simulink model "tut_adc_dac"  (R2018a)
settings: Solver=VariableStepAuto  StartTime=0.0  StopTime=10.0  RelTol=1e-3
undefined symbols (not defined in the file): adc_data_ch1, adc_data_ch2, adc_data_valid, Bit, Both, bram, c, d, hex2dec, led, Location, Lower, Minimum_Area, out, RED_PITAYA_10, reg, ROACH, ROACH2, rst_cntrl, Unsigned, Upper, Width, xc7z010
libraries: xbsIndex_r4 x149, xps_library x6, casper_library_misc x2
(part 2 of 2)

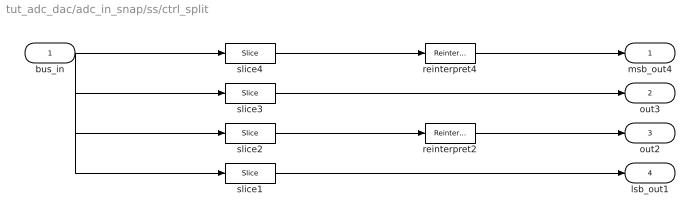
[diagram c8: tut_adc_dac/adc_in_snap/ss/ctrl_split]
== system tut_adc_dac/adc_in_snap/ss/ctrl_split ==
  bus_in : Inport
  reinterpret2 : xbsIndex_r4/Reinterpret  force_arith_type=on  arith_type=Unsigned  force_bin_pt=on  bin_pt=0  block_type=reinterpret
  reinterpret4 : xbsIndex_r4/Reinterpret  force_arith_type=on  arith_type=Unsigned  force_bin_pt=on  bin_pt=0  block_type=reinterpret
  slice1 : xbsIndex_r4/Slice  nbits=1  boolean_output=on  mode=Upper Bit Location + Width  bit1=-31  base1=MSB of Input  bit0=0  base0=LSB of Input  dbl_ovrd=off  block_type=slice
  slice2 : xbsIndex_r4/Slice  nbits=2  boolean_output=off  mode=Upper Bit Location + Width  bit1=-29  base1=MSB of Input  bit0=0  base0=LSB of Input  dbl_ovrd=off  block_type=slice
  slice3 : xbsIndex_r4/Slice  nbits=1  boolean_output=on  mode=Upper Bit Location + Width  bit1=-28  base1=MSB of Input  bit0=0  base0=LSB of Input  dbl_ovrd=off  block_type=slice
  slice4 : xbsIndex_r4/Slice  nbits=28  boolean_output=off  mode=Upper Bit Location + Width  bit1=0  base1=MSB of Input  bit0=0  base0=LSB of Input  dbl_ovrd=off  block_type=slice
  msb_out4 : Outport
  out3 : Outport  Port=2
  out2 : Outport  Port=3
  lsb_out1 : Outport  Port=4
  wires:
  bus_in/1 -> slice4/1, slice3/1, slice2/1, slice1/1
  slice4/1 -> reinterpret4/1
  reinterpret4/1 -> msb_out4/1
  slice3/1 -> out3/1
  slice2/1 -> reinterpret2/1
  reinterpret2/1 -> out2/1
  slice1/1 -> lsb_out1/1

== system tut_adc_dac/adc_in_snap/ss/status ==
  out_reg : Inport
  assert_reg : xbsIndex_r4/Assert  assert_type=on  type_source=Explicitly  gui_display_data_type=Fixed-point  arith_type=Unsigned  n_bits=32  bin_pt=0  preci_type=Single  exp_width=8  frac_width=24  assert_rate=off  rate_source=Explicitly  period=1  output_port=on  block_type=assert
  cast_gw : xbsIndex_r4/Convert  gui_display_data_type=Fixed-point  arith_type=Unsigned  n_bits=32  bin_pt=0  float_type=Single  exp_bits=8  fraction_bits=24  quantization=Truncate  overflow=Wrap  en=off  latency=1  pipeline=off  dbl_ovrd=off  block_type=convert
  io_delay : xbsIndex_r4/Delay  rst=off  infoeditControl=Selection of Reset will increase slice count due to use of real FFs and instead of SRLs  en=off  latency=0  reg_retiming=on  dbl_ovrd=off  block_type=delay
  reint1 : xbsIndex_r4/Reinterpret  force_arith_type=on  arith_type=Unsigned  force_bin_pt=on  bin_pt=0  block_type=reinterpret
  sim_out : Terminator
  tut_adc_dac_adc_in_snap_ss_status_user_data_in : xbsIndex_r4/Gateway Out  inherit_from_input=off  hdl_port=on  rows=1  columns=1  UseAsDAC=off  DACChannel='1'  interface=None  automatic_assignment=on  address_offset=hex2dec('00')  intf_name=''  intf_description=''  timing_constraint=None  locs_specified=off  LOCs={}  io_standard={}  block_type=gatewayout
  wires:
  io_delay/1 -> cast_gw/1
  cast_gw/1 -> tut_adc_dac_adc_in_snap_ss_status_user_data_in/1
  tut_adc_dac_adc_in_snap_ss_status_user_data_in/1 -> sim_out/1
  out_reg/1 -> assert_reg/1
  assert_reg/1 -> reint1/1
  reint1/1 -> io_delay/1

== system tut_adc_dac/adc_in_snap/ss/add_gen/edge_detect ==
  in : Inport
  Delay : xbsIndex_r4/Delay  rst=off  infoeditControl=Selection of Reset will increase slice count due to use of real FFs and instead of SRLs  en=off  latency=1  reg_retiming=off  dbl_ovrd=off  block_type=delay
  Inverter : xbsIndex_r4/Inverter  en=off  latency=0  dbl_ovrd=off  block_type=inv
  edge_op : xbsIndex_r4/Logical  logical_function=XNOR  inputs=2  en=off  latency=0  precision=Full  arith_type=Unsigned  n_bits=8  bin_pt=2  align_bp=on  dbl_ovrd=off  block_type=logical
  out : Outport
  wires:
  Delay/1 -> edge_op/2
  in/1 -> Delay/1, Inverter/1
  edge_op/1 -> out/1
  Inverter/1 -> edge_op/1

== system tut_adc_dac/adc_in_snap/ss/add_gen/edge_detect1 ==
  in : Inport
  Delay : xbsIndex_r4/Delay  rst=off  infoeditControl=Selection of Reset will increase slice count due to use of real FFs and instead of SRLs  en=off  latency=1  reg_retiming=off  dbl_ovrd=off  block_type=delay
  Inverter : xbsIndex_r4/Inverter  en=off  latency=0  dbl_ovrd=off  block_type=inv
  edge_op : xbsIndex_r4/Logical  logical_function=XNOR  inputs=2  en=off  latency=0  precision=Full  arith_type=Unsigned  n_bits=8  bin_pt=2  align_bp=on  dbl_ovrd=off  block_type=logical
  out : Outport
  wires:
  Inverter/1 -> edge_op/1
  edge_op/1 -> out/1
  in/1 -> Inverter/1, Delay/1
  Delay/1 -> edge_op/2

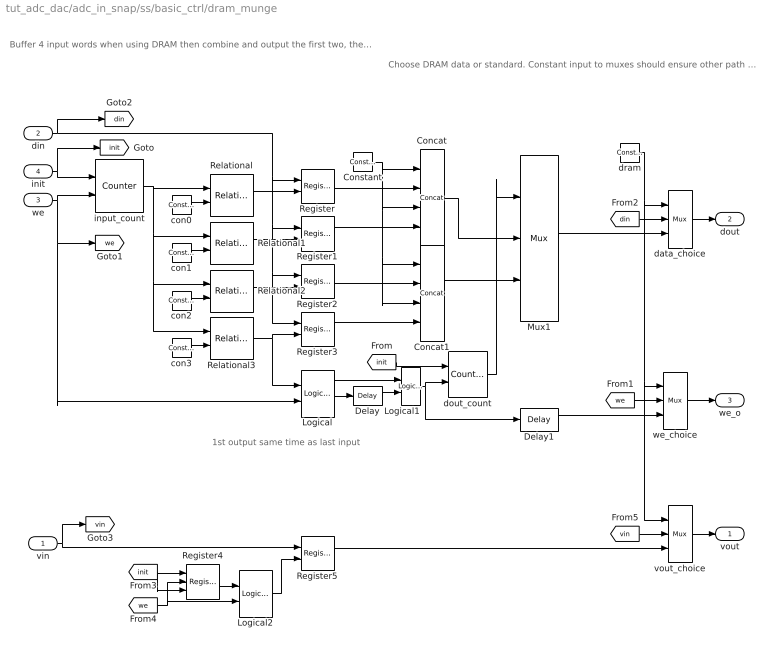
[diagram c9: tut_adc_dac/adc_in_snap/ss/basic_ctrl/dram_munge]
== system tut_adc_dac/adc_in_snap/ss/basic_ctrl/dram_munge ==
  note: 1st output same time as last input
  note: Choose DRAM data or standard. Constant input to muxes should ensure other path optimised away
  note: Buffer 4 input words when using DRAM then combine and output the first two, then second. Ensures that a full burst goes through every time so that status register records number of bytes fully in DRAM
  vin : Inport
  din : Inport  Port=2
  we : Inport  Port=3
  init : Inport  Port=4
  Concat : xbsIndex_r4/Concat  num_inputs=4  dbl_ovrd=off  block_type=concat
  Concat1 : xbsIndex_r4/Concat  num_inputs=4  dbl_ovrd=off  block_type=concat
  Constant : xbsIndex_r4/Constant  const=0  gui_display_data_type=Fixed-point  arith_type=Unsigned  n_bits=8  bin_pt=0  preci_type=Single  exp_width=8  frac_width=24  explicit_period=on  period=1  equ=P=C  opselect=C  inp2=PCIN>>17  opr=+  inp1=P  carry=CIN  dbl_ovrd=off  block_type=constant
  Delay : xbsIndex_r4/Delay  rst=off  infoeditControl=Selection of Reset will increase slice count due to use of real FFs and instead of SRLs  en=off  latency=1  reg_retiming=off  dbl_ovrd=off  block_type=delay
  Delay1 : xbsIndex_r4/Delay  rst=off  infoeditControl=Selection of Reset will increase slice count due to use of real FFs and instead of SRLs  en=off  latency=1  reg_retiming=off  dbl_ovrd=off  block_type=delay
  Logical : xbsIndex_r4/Logical  logical_function=AND  inputs=2  en=off  latency=1  precision=Full  arith_type=Unsigned  n_bits=16  bin_pt=0  align_bp=on  dbl_ovrd=off  block_type=logical
  Logical1 : xbsIndex_r4/Logical  logical_function=OR  inputs=2  en=off  latency=0  precision=Full  arith_type=Unsigned  n_bits=16  bin_pt=0  align_bp=on  dbl_ovrd=off  block_type=logical
  Logical2 : xbsIndex_r4/Logical  logical_function=AND  inputs=2  en=off  latency=0  precision=Full  arith_type=Unsigned  n_bits=16  bin_pt=0  align_bp=on  dbl_ovrd=off  block_type=logical
  Mux1 : xbsIndex_r4/Mux  inputs=2  en=off  latency=1  precision=Full  arith_type=Unsigned  n_bits=16  bin_pt=14  quantization=Truncate  overflow=Wrap  dbl_ovrd=off  block_type=mux
  Register{,1..3,5} (5 alike) : xbsIndex_r4/Register  init=0  rst=off  en=on  dbl_ovrd=off  block_type=register
  Register4 : xbsIndex_r4/Register  init=0  rst=on  en=on  dbl_ovrd=off  block_type=register
  Relational{,1..3} (4 alike) : xbsIndex_r4/Relational  mode=a=b  op_type=Bool  en=off  latency=0  dbl_ovrd=off  block_type=relational
  con0 : xbsIndex_r4/Constant  const=0  gui_display_data_type=Fixed-point  arith_type=Unsigned  n_bits=2  bin_pt=0  preci_type=Single  exp_width=8  frac_width=24  explicit_period=on  period=1  equ=P=C  opselect=C  inp2=PCIN>>17  opr=+  inp1=P  carry=CIN  dbl_ovrd=off  block_type=constant
  con1 : xbsIndex_r4/Constant  const=1  gui_display_data_type=Fixed-point  arith_type=Unsigned  n_bits=2  bin_pt=0  preci_type=Single  exp_width=8  frac_width=24  explicit_period=on  period=1  equ=P=C  opselect=C  inp2=PCIN>>17  opr=+  inp1=P  carry=CIN  dbl_ovrd=off  block_type=constant
  con2 : xbsIndex_r4/Constant  const=2  gui_display_data_type=Fixed-point  arith_type=Unsigned  n_bits=2  bin_pt=0  preci_type=Single  exp_width=8  frac_width=24  explicit_period=on  period=1  equ=P=C  opselect=C  inp2=PCIN>>17  opr=+  inp1=P  carry=CIN  dbl_ovrd=off  block_type=constant
  con3 : xbsIndex_r4/Constant  const=3  gui_display_data_type=Fixed-point  arith_type=Unsigned  n_bits=2  bin_pt=0  preci_type=Single  exp_width=8  frac_width=24  explicit_period=on  period=1  equ=P=C  opselect=C  inp2=PCIN>>17  opr=+  inp1=P  carry=CIN  dbl_ovrd=off  block_type=constant
  data_choice : xbsIndex_r4/Mux  inputs=2  en=off  latency=0  precision=User Defined  arith_type=Unsigned  n_bits=32  bin_pt=0  quantization=Truncate  overflow=Wrap  dbl_ovrd=off  block_type=mux
  dout_count : xbsIndex_r4/Counter  cnt_type=Free Running  cnt_to=Inf  operation=Up  start_count=0  cnt_by_val=1  arith_type=Unsigned  n_bits=1  bin_pt=0  load_pin=off  rst=on  en=on  explicit_period=on  period=1  use_behavioral_HDL=off  implementation=Fabric  dbl_ovrd=off  block_type=counter
  dram : xbsIndex_r4/Constant  const=0  gui_display_data_type=Fixed-point  arith_type=Boolean  n_bits=16  bin_pt=14  preci_type=Single  exp_width=8  frac_width=24  explicit_period=on  period=1  equ=P=C  opselect=C  inp2=PCIN>>17  opr=+  inp1=P  carry=CIN  dbl_ovrd=off  block_type=constant
  input_count : xbsIndex_r4/Counter  cnt_type=Free Running  cnt_to=Inf  operation=Up  start_count=0  cnt_by_val=1  arith_type=Unsigned  n_bits=2  bin_pt=0  load_pin=off  rst=on  en=on  explicit_period=on  period=1  use_behavioral_HDL=off  implementation=Fabric  dbl_ovrd=off  block_type=counter
  vout_choice : xbsIndex_r4/Mux  inputs=2  en=off  latency=0  precision=Full  arith_type=Unsigned  n_bits=16  bin_pt=14  quantization=Truncate  overflow=Wrap  dbl_ovrd=off  block_type=mux
  we_choice : xbsIndex_r4/Mux  inputs=2  en=off  latency=0  precision=Full  arith_type=Unsigned  n_bits=16  bin_pt=14  quantization=Truncate  overflow=Wrap  dbl_ovrd=off  block_type=mux
  vout : Outport
  dout : Outport  Port=2
  we_o : Outport  Port=3
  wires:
  Register3/1 -> Concat1/4
  Register2/1 -> Concat1/2
  Constant/1 -> Concat1/3, Concat1/1, Concat/3, Concat/1
  Register1/1 -> Concat/4
  Register/1 -> Concat/2
  [vin] -> vout_choice/2
  Register5/1 -> vout_choice/3
  vout_choice/1 -> vout/1
  Logical2/1 -> Register5/2
  [we] -> Logical2/2, Register4/2
  vin/1 -> [vin], Register5/1
  Register4/1 -> Logical2/1
  [init] -> Register4/3, Register4/1
  dram/1 -> vout_choice/1, we_choice/1, data_choice/1
  [din] -> data_choice/2
  Mux1/1 -> data_choice/3
  [we] -> we_choice/2
  Delay1/1 -> we_choice/3
  we_choice/1 -> we_o/1
  dout_count/1 -> Mux1/1
  [init] -> dout_count/1
  Logical1/1 -> Delay1/1, dout_count/2
  Concat1/1 -> Mux1/3
  Concat/1 -> Mux1/2
  Delay/1 -> Logical1/2
  Logical/1 -> Logical1/1, Delay/1
  Relational3/1 -> Logical/1, Register3/2
  Relational2/1 -> Register2/2
  Relational1/1 -> Register1/2
  Relational/1 -> Register/2
  con3/1 -> Relational3/2
  con2/1 -> Relational2/2
  con1/1 -> Relational1/2
  con0/1 -> Relational/2
  input_count/1 -> Relational3/1, Relational2/1, Relational1/1, Relational/1
  din/1 -> [din], Register3/1, Register2/1, Register1/1, Register/1
  we/1 -> [we], Logical/2, input_count/2
  init/1 -> [init], input_count/1
  data_choice/1 -> dout/1

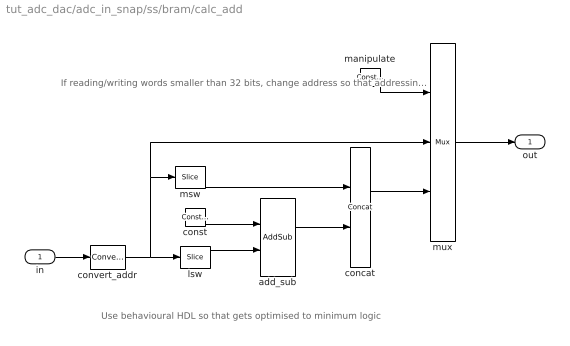
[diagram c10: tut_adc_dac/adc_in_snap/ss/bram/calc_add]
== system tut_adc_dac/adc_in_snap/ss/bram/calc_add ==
  note: If reading/writing words smaller than 32 bits, change address so that addressing is big endian instead of little, otherwise pass through
  note: Use behavioural HDL so that gets optimised to minimum logic
  in : Inport
  add_sub : xbsIndex_r4/AddSub  mode=Subtraction  use_carryin=off  use_carryout=off  en=off  latency=0  precision=User Defined  arith_type=Unsigned  n_bits=max(1, log2(32/data_width))  bin_pt=0  quantization=Truncate  overflow=Wrap  use_behavioral_HDL=on  hw_selection=Fabric  pipelined=off  dbl_ovrd=off  block_type=addsub
  concat : xbsIndex_r4/Concat  num_inputs=2  dbl_ovrd=off  block_type=concat
  const : xbsIndex_r4/Constant  const=max(0, 32/data_width-1)  gui_display_data_type=Fixed-point  arith_type=Unsigned  n_bits=max(1, log2(32/data_width))  bin_pt=0  preci_type=Single  exp_width=8  frac_width=24  explicit_period=on  period=sample_rate  equ=P=C  opselect=C  inp2=PCIN>>17  opr=+  inp1=P  carry=CIN  dbl_ovrd=off  block_type=constant
  convert_addr : xbsIndex_r4/Convert  gui_display_data_type=Fixed-point  arith_type=Unsigned  n_bits=addr_width  bin_pt=0  float_type=Single  exp_bits=8  fraction_bits=24  quantization=Truncate  overflow=Wrap  en=off  latency=0  pipeline=off  dbl_ovrd=off  block_type=convert
  lsw : xbsIndex_r4/Slice  nbits=max(1, log2(32/data_width))  boolean_output=off  mode=Lower Bit Location + Width  bit1=0  base1=MSB of Input  bit0=0  base0=LSB of Input  dbl_ovrd=off  block_type=slice
  manipulate : xbsIndex_r4/Constant  const=min(1, floor(32/data_width) - 1)  gui_display_data_type=Fixed-point  arith_type=Unsigned  n_bits=1  bin_pt=0  preci_type=Single  exp_width=8  frac_width=24  explicit_period=on  period=sample_rate  equ=P=C  opselect=C  inp2=PCIN>>17  opr=+  inp1=P  carry=CIN  dbl_ovrd=off  block_type=constant
  msw : xbsIndex_r4/Slice  nbits=addr_width - max(1, log2(32/data_width))  boolean_output=off  mode=Upper Bit Location + Width  bit1=0  base1=MSB of Input  bit0=0  base0=LSB of Input  dbl_ovrd=off  block_type=slice
  mux : xbsIndex_r4/Mux  inputs=2  en=off  latency=0  precision=Full  arith_type=Unsigned  n_bits=16  bin_pt=14  quantization=Truncate  overflow=Wrap  dbl_ovrd=off  block_type=mux
  out : Outport
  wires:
  in/1 -> convert_addr/1
  add_sub/1 -> concat/2
  msw/1 -> concat/1
  concat/1 -> mux/3
  manipulate/1 -> mux/1
  mux/1 -> out/1
  lsw/1 -> add_sub/2
  const/1 -> add_sub/1
  convert_addr/1 -> lsw/1, msw/1, mux/2

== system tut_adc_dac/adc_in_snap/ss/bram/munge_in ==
  din : Inport
  reinterpret_out : xbsIndex_r4/Reinterpret  force_arith_type=on  arith_type=Unsigned  force_bin_pt=on  bin_pt=0  block_type=reinterpret
  dout : Outport
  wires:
  reinterpret_out/1 -> dout/1
  din/1 -> reinterpret_out/1

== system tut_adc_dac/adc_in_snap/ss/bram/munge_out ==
  din : Inport
  reinterpret_out : xbsIndex_r4/Reinterpret  force_arith_type=on  arith_type=Unsigned  force_bin_pt=on  bin_pt=0  block_type=reinterpret
  dout : Outport
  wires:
  reinterpret_out/1 -> dout/1
  din/1 -> reinterpret_out/1

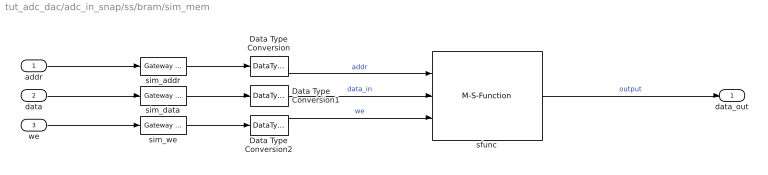
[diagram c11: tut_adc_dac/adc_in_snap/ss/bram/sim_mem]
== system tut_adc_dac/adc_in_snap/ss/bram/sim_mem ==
  addr : Inport
  data : Inport  Port=2
  we : Inport  Port=3
  Data Type Conversion : DataTypeConversion  OutDataTypeStr=single
  Data Type Conversion1 : DataTypeConversion  OutDataTypeStr=double
  Data Type Conversion2 : DataTypeConversion  OutDataTypeStr=boolean
  sfunc : M-S-Function  FunctionName=shared_bram_sim_sfunc  Parameters=depth_bits, latency, init_vals  mask{depth_bits=addr_width, latency=csp_latency, init_vals=init_vals}
      mask prompts: depth_bits "Depth (2^?):"; latency "Latency (>=1):"; init_vals "Initial values:"
  sim_addr : xbsIndex_r4/Gateway Out  inherit_from_input=off  hdl_port=off  rows=1  columns=1  UseAsDAC=off  DACChannel='1'  interface=None  automatic_assignment=on  address_offset=hex2dec('00')  intf_name=''  intf_description=''  timing_constraint=None  locs_specified=off  LOCs={}  io_standard={}  block_type=gatewayout
  sim_data : xbsIndex_r4/Gateway Out  inherit_from_input=off  hdl_port=off  rows=1  columns=1  UseAsDAC=off  DACChannel='1'  interface=None  automatic_assignment=on  address_offset=hex2dec('00')  intf_name=''  intf_description=''  timing_constraint=None  locs_specified=off  LOCs={}  io_standard={}  block_type=gatewayout
  sim_we : xbsIndex_r4/Gateway Out  inherit_from_input=off  hdl_port=off  rows=1  columns=1  UseAsDAC=off  DACChannel='1'  interface=None  automatic_assignment=on  address_offset=hex2dec('00')  intf_name=''  intf_description=''  timing_constraint=None  locs_specified=off  LOCs={}  io_standard={}  block_type=gatewayout
  data_out : Outport
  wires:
  addr/1 -> sim_addr/1
  data/1 -> sim_data/1
  we/1 -> sim_we/1
  sim_addr/1 -> Data Type Conversion/1
  sim_data/1 -> Data Type Conversion1/1
  sim_we/1 -> Data Type Conversion2/1
  Data Type Conversion/1 -> sfunc/1  "addr"
  Data Type Conversion1/1 -> sfunc/2  "data_in"
  Data Type Conversion2/1 -> sfunc/3  "we"
  sfunc/1 -> data_out/1  "output"
